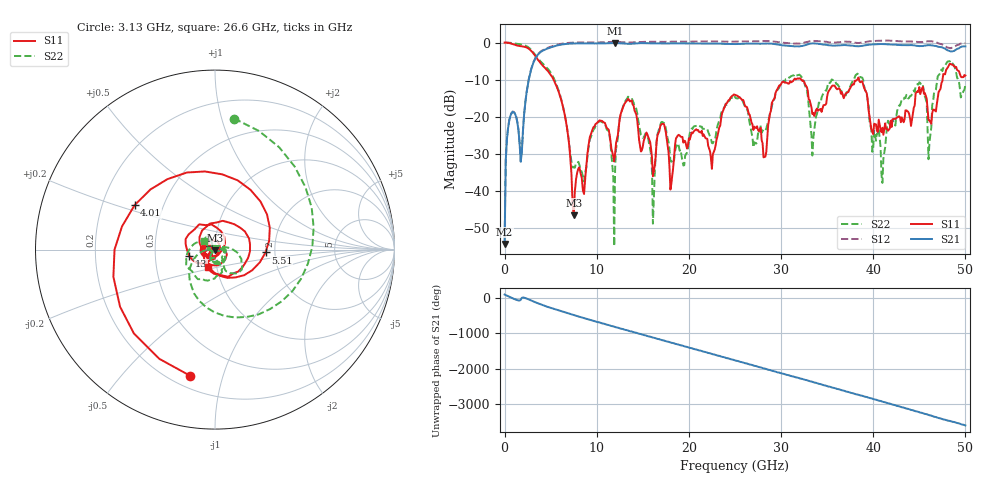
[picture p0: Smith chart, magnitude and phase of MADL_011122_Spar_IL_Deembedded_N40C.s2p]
#	HZ	S	DB	R	50
!Frequency	S11 (dB)	S11-Ang	S21 Deemb (dB)	S21-Ang	S12 Deemb (dB)	S12-Ang	S22 (dB)	S22-Ang
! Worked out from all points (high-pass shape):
!   401 points, 10 MHz to 50 GHz, reference 50 ohm
!   highest |S21| = -0.11 dB at 12 GHz (marker M1); lowest = -54.4 dB at 10 MHz (marker M2)
!   |S21| within 3 dB of the highest: 3.663 GHz to end of sweep
!   lowest |S11| = -46.7 dB at 7.51 GHz (marker M3), VSWR 1.01, Z = 50.3 - j0.383 ohm
!   |S11| at or under -10 dB: 5.324 GHz to 31.4 GHz (26.08 GHz wide, 142 % of centre); 32.2 GHz to 38.27 GHz (6.071 GHz wide, 17.2 % of centre); 38.46 GHz to 47.52 GHz (9.062 GHz wide, 21.1 % of centre)
!   |S22| runs from -55.0 to 0.0 dB; largest |S21 - S12| = 0.13
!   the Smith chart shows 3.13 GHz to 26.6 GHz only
!   S11 on the Smith chart (normalised r, x): 3.13 GHz: 0.27, -0.79; 4.01 GHz: 0.34, +0.23; 5.51 GHz: 1.78, -0.06; 13 GHz: 0.75, -0.05; 26.6 GHz: 0.91, -0.18
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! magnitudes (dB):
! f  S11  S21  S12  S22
! 10 MHz  0.0  -54.4  -52.8  0.0
! 510 MHz  -0.1  -21.1  -21.0  0.0
! 1.76 GHz  -0.9  -32.2  -32.0  -0.4
! 3.13 GHz  -2.9  -5.4  -5.3  -2.6
! 4.01 GHz  -5.8  -2.4  -2.2  -5.3
! 5.51 GHz  -11.0  -0.9  -0.7  -10.5
! 7.51 GHz  -46.7  -0.2  0.0  -33.7
! 8.38 GHz  -36.5  -0.2  0.1  -34.9
! 10.4 GHz  -21.1  -0.2  0.1  -21.3
! 12 GHz  -29.9  -0.1  0.2  -34.0
! 13 GHz  -16.6  -0.3  0.1  -16.1
! 16.1 GHz  -36.1  -0.2  0.3  -48.9
! 16.8 GHz  -23.9  -0.2  0.2  -23.1
! 22.5 GHz  -34.1  -0.2  0.4  -27.1
! 25.1 GHz  -14.2  -0.4  0.3  -15.0
! 26.6 GHz  -19.5  -0.2  0.4  -21.8
! 31.8 GHz  -9.6  -1.0  -0.2  -8.8
! 33.4 GHz  -19.3  -0.2  0.5  -30.5
! 38.3 GHz  -9.9  -1.0  -0.1  -8.4
! 41 GHz  -23.0  -0.4  0.6  -37.9
! 41.8 GHz  -23.2  -0.5  0.5  -22.2
! 50 GHz  -8.9  -1.0  -0.1  -11.3
